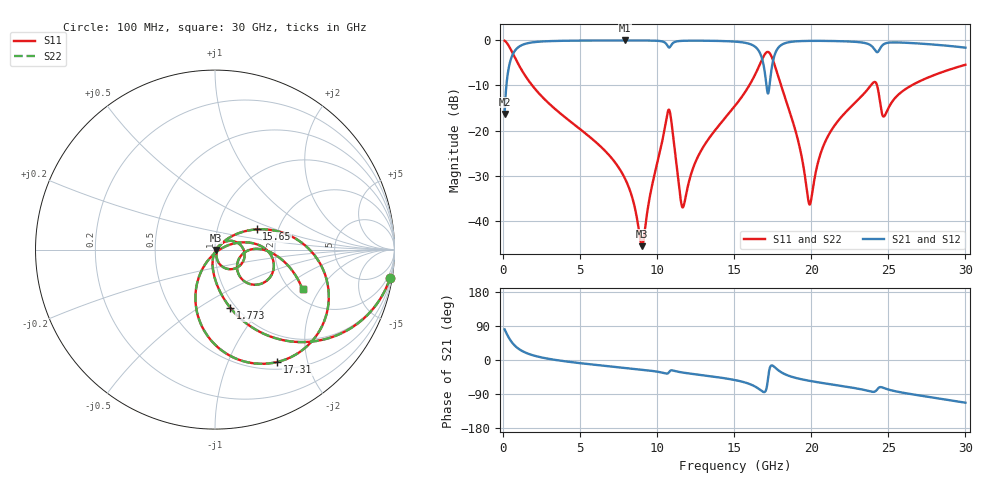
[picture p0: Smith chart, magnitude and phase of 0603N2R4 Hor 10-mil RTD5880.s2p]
# GHz S MA R 50
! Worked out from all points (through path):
!   3201 points, 100 MHz to 30 GHz, reference 50 ohm
!   highest |S21| = -0.04 dB at 7.893 GHz (marker M1); lowest = -16.3 dB at 100 MHz (marker M2)
!   group delay of S21, straight-line fit = 11.4 ps
!   lowest |S11| = -45.6 dB at 9.014 GHz (marker M3), VSWR 1.01, Z = 50.5 - j0.256 ohm
!   |S11| at or under -10 dB: 1.89 GHz to 15.98 GHz (14.09 GHz wide, 158 % of centre); 18.04 GHz to 23.86 GHz (5.82 GHz wide, 27.8 % of centre); 24.27 GHz to 26.51 GHz (2.237 GHz wide, 8.81 % of centre)
!   |S22| runs from -45.6 to -0.1 dB; largest |S21 - S12| = 0
!   S11 on the Smith chart (normalised r, x): 100 MHz: 1, -13; 1.773 GHz: 0.94, -0.69; 15.65 GHz: 1.55, +0.37; 17.31 GHz: 0.60, -1.53; 30 GHz: 2.29, -1.42
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0.1  0.9882 -9.1  0.1529 80.9  0.1529 80.9  0.9882 -9.1
0.6045625  0.7291 -44.9  0.6837 45.1  0.6837 45.1  0.7291 -44.9
1.772531  0.3358 -75.2  0.9405 14.5  0.9405 14.5  0.3358 -75.2
5.089563  0.1007 -97.2  0.9922 -8.8  0.9922 -8.8  0.1007 -97.2
7.892688  0.02977 -103.2  0.9955 -20.8  0.9955 -20.8  0.02977 -103.2
9.013938  0.00523 -29.0  0.9947 -25.6  0.9947 -25.6  0.00523 -29.0
10.06978  0.04848 42.7  0.9853 -31.2  0.9853 -31.2  0.04848 42.7
10.78925  0.1682 -28.1  0.8318 -31.0  0.8318 -31.0  0.1682 -28.1
11.68625  0.01419 -12.0  0.9866 -33.3  0.9866 -33.3  0.01419 -12.0
12.75144  0.05574 41.9  0.9896 -39.1  0.9896 -39.1  0.05574 41.9
15.05  0.1875 32.3  0.9666 -53.0  0.9666 -53.0  0.1875 32.3
15.648  0.2581 25.9  0.9418 -58.7  0.9418 -58.7  0.2581 25.9
16.60106  0.5121 1.6  0.7592 -76.4  0.7592 -76.4  0.5121 1.6
17.00284  0.7067 -27.0  0.4177 -83.6  0.4177 -83.6  0.7067 -27.0
17.31119  0.7159 -61.0  0.3406 -20.5  0.3406 -20.5  0.7159 -61.0
17.93722  0.3596 -106.3  0.8552 -29.4  0.8552 -29.4  0.3596 -106.3
20.03956  0.01921 -15.3  0.9851 -56.1  0.9851 -56.1  0.01921 -15.3
20.74969  0.06519 17.5  0.9846 -60.9  0.9846 -60.9  0.06519 17.5
22.01109  0.1453 15.8  0.9756 -68.8  0.9756 -68.8  0.1453 15.8
24.06672  0.3437 -18.2  0.8083 -84.0  0.8083 -84.0  0.3437 -18.2
25.01978  0.1793 -2.2  0.9408 -78.1  0.9408 -78.1  0.1793 -2.2
30  0.5353 -24.4  0.8284 -112.7  0.8284 -112.7  0.5353 -24.4
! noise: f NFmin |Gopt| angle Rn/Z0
0.1  0.0004225  0.9448  0.905  0.001714
3.417  0.004007  0.8088  9.999  0.004331
6.743  0.006987  0.7872  19.31  0.00657
10.06  0.01699  0.8649  28.49  0.02537
13.39  0.01611  0.8173  37.58  0.01656
16.7  0.08285  0.9529  46.58  0.3341
20.03  0.02474  0.8257  55.38  0.02346
23.35  0.03691  0.8631  63.74  0.04178
26.67  0.03083  0.8199  71.82  0.02365
30  0.0339  0.8189  79.57  0.02332
